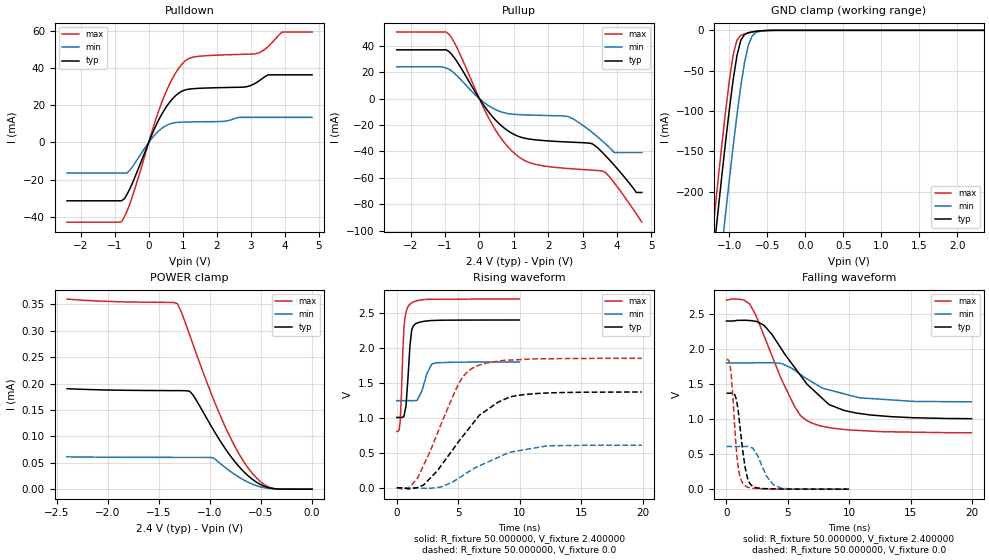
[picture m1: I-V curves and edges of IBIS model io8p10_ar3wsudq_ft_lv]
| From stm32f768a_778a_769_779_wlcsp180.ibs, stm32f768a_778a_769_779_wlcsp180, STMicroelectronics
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|   Model io8p10_ar3wsudq_ft_lv
[Model]  io8p10_ar3wsudq_ft_lv
Model_type I/O
Polarity   Non-Inverting
Enable   Active-Low
Vinl =   0.720000V
Vinh =   1.680000V
Vmeas =  1.200000V
Cref =   40.000000pF
Rref =   100.000000M
Vref =   0.0V
C_comp   3.720900pF   3.684200pF   3.822900pF
[Temperature Range]   25.000000   0.125000k   -40.000000
[Pullup Reference]   2.400000V   1.800000V   2.700000V
[Pulldown Reference]   0.0V   0.0V   0.0V
[POWER Clamp Reference]   2.400000V   1.800000V   2.700000V
[GND Clamp Reference]   0.0V   0.0V   0.0V
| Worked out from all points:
|   slope of the pulldown table from 0 to 0.36 V, typ, clamps not added: 25 ohm
|   slope of the pullup table from 0 to 0.36 V, typ, clamps not added: 27.7 ohm
|   GND clamp passes 1 mA (typ) near -0.62 V on its own axis
|   rising waveform, R_fixture 50.000000, V_fixture 2.400000: 20-80 % time 334ps typ, 652ps min, 263ps max; typ from 1.01 V to 2.4 V
|   rising waveform, R_fixture 50.000000, V_fixture 0.0: 20-80 % time 3.76ns typ, 4.01ns min, 2.7ns max; typ from 0 V to 1.37 V
|   falling waveform, R_fixture 50.000000, V_fixture 2.400000: 20-80 % time 3.84ns typ, 4.04ns min, 2.77ns max; typ from 2.4 V to 1.01 V
|   falling waveform, R_fixture 50.000000, V_fixture 0.0: 20-80 % time 591ps typ, 1.03ns min, 463ps max; typ from 1.37 V to 0 V
[Pulldown]
|Voltage   I(typ)   I(min)   I(max)
-2.4V     -31.47mA   -16.45mA   -43.01mA
-800mV    -31.47mA   -16.45mA   -42.85mA
-480mV    -21.98mA   -13.17mA   -29.21mA
80mV      3.63mA     1.966mA    5.014mA
480mV     18.16mA    8.738mA    26.02mA
800mV     25.38mA    10.72mA    37.77mA
1.12V     28.53mA    11.02mA    44.6mA
2.8V      29.84mA    13.51mA    47.53mA
3.2V      32.66mA    13.51mA    48.04mA
3.52V     36.44mA    13.51mA    51.84mA
3.92V     36.44mA    13.51mA    59.5mA
4.8V      36.44mA    13.51mA    59.5mA
[Pullup]
|Voltage   I(typ)   I(min)   I(max)
-2.4V     36.92mA    24.04mA    50.36mA
-960mV    36.92mA    23.05mA    50.36mA
-640mV    27.65mA    17.04mA    37.98mA
320mV     -11.75mA   -6.207mA   -17.08mA
960mV     -26.47mA   -11.82mA   -40.02mA
1.52V     -30.88mA   -12.51mA   -49.05mA
2.56V     -32.88mA   -13.52mA   -52.9mA
3.28V     -34.25mA   -25.64mA   -54.18mA
3.6V      -41.44mA   -32.74mA   -55.03mA
3.92V     -50.46mA   -40.9mA    -63.79mA
4.56V     -71.1mA    -40.9mA    -87.26mA
4.72V     -71.1mA    -40.9mA    -93.6mA
[GND_clamp]
|Voltage   I(typ)   I(min)   I(max)
-2.4V     -1.43A     -1.515A    -1.399A
-1.25V    -315.9mA   -407.2mA   -278.2mA
-1.2V     -270.1mA   -361.3mA   -232.1mA
-1.15V    -225mA     -316mA     -186.8mA
-1.1V     -180.9mA   -271.3mA   -142.7mA
-1.05V    -138.2mA   -227.5mA   -100.5mA
-950mV    -61.14mA   -143.6mA   -30.43mA
-900mV    -31.23mA   -104.7mA   -12.14mA
-850mV    -12.49mA   -69.4mA    -6.221mA
-750mV    -2.898mA   -18.35mA   -3.18mA
-600mV    -750.2uA   -1.218mA   -738.3uA
2.35V     0A         0A         0A
[POWER_clamp]
|Voltage   I(typ)   I(min)   I(max)
-2.4V     190.2uA    61.19uA    359.9uA
-1.32V    186.6uA    60.14uA    351.2uA
-1.29V    186.5uA    60.13uA    339.6uA
-1.2V     185.4uA    60.11uA    292.6uA
-1.17V    179.2uA    60.11uA    276.3uA
-960mV    110.2uA    58.62uA    167.5uA
-870mV    82.44uA    43.99uA    126.3uA
-750mV    50.58uA    26.92uA    78.64uA
-630mV    25.94uA    13.41uA    41.02uA
-510mV    9.22uA     4.527uA    14.97uA
-420mV    2.425uA    1.38uA     3.75uA
0V        0A         0A         0A
[Ramp]
| variable   typ   min   max
dV/dt_r  0.82206/3.76189n   0.36570/4.00648n   1.11348/2.70300n
dV/dt_f  0.83262/3.83766n   0.33192/4.09052n   1.13642/2.77245n
R_load = 50.000000
[Rising Waveform]
R_fixture= 50.000000
V_fixture= 2.400000
V_fixture_min= 1.800000
V_fixture_max= 2.700000
|time   V(typ)   V(min)   V(max)
0s        1.006V     1.247V     804.8mV
200.2ps   1.006V     1.247V     830.4mV
280.3ps   1.006V     1.247V     952.2mV
580.6ps   1.019V     1.247V     2.262V
760.8ps   1.193V     1.247V     2.51V
1.021ns   1.88V      1.247V     2.617V
1.241ns   2.271V     1.246V     2.647V
1.762ns   2.363V     1.286V     2.682V
2.863ns   2.393V     1.769V     2.696V
9.97ns    2.4V       1.8V       2.699V
[Rising Waveform]
R_fixture= 50.000000
V_fixture= 0.0
V_fixture_min= 0.0
V_fixture_max= 0.0
|time   V(typ)   V(min)   V(max)
0s        159.6uV    64.29uV    111.4uV
1.081ns   -14.23mV   123.7uV    11.59mV
1.682ns   3.867mV    -934uV     138.3mV
3.283ns   240mV      2.908mV    767.8mV
5.005ns   653.1mV    133.4mV    1.479V
6.286ns   940.4mV    278mV      1.723V
8.248ns   1.225V     434.9mV    1.811V
9.57ns    1.312V     519.2mV    1.83V
12.25ns   1.356V     601mV      1.846V
19.94ns   1.37V      609mV      1.851V
[Falling Waveform]
R_fixture= 50.000000
V_fixture= 2.400000
V_fixture_min= 1.800000
V_fixture_max= 2.700000
|time   V(typ)   V(min)   V(max)
0s        2.4V       1.8V       2.699V
1.401ns   2.41V      1.8V       2.701V
1.882ns   2.407V     1.801V     2.644V
3.083ns   2.334V     1.805V     2.178V
4.484ns   1.998V     1.793V     1.565V
5.526ns   1.742V     1.699V     1.186V
6.687ns   1.477V     1.561V     965.1mV
8.328ns   1.21V      1.417V     879.6mV
10.53ns   1.087V     1.317V     839.8mV
19.94ns   1.006V     1.247V     804.8mV
[Falling Waveform]
R_fixture= 50.000000
V_fixture= 0.0
V_fixture_min= 0.0
V_fixture_max= 0.0
|time   V(typ)   V(min)   V(max)
0s        1.37V      609mV      1.851V
320.3ps   1.37V      609mV      1.736V
820.8ps   1.271V     608.9mV    539.8mV
1.061ns   955.5mV    608.6mV    208.2mV
1.421ns   431.1mV    609.2mV    65.34mV
1.702ns   164.6mV    608.6mV    31.01mV
2.062ns   51.7mV     591.9mV    14.99mV
3.283ns   5.812mV    180.7mV    2.916mV
4.464ns   1.861mV    14.2mV     843.2uV
9.97ns    159.6uV    64.29uV    111.4uV
